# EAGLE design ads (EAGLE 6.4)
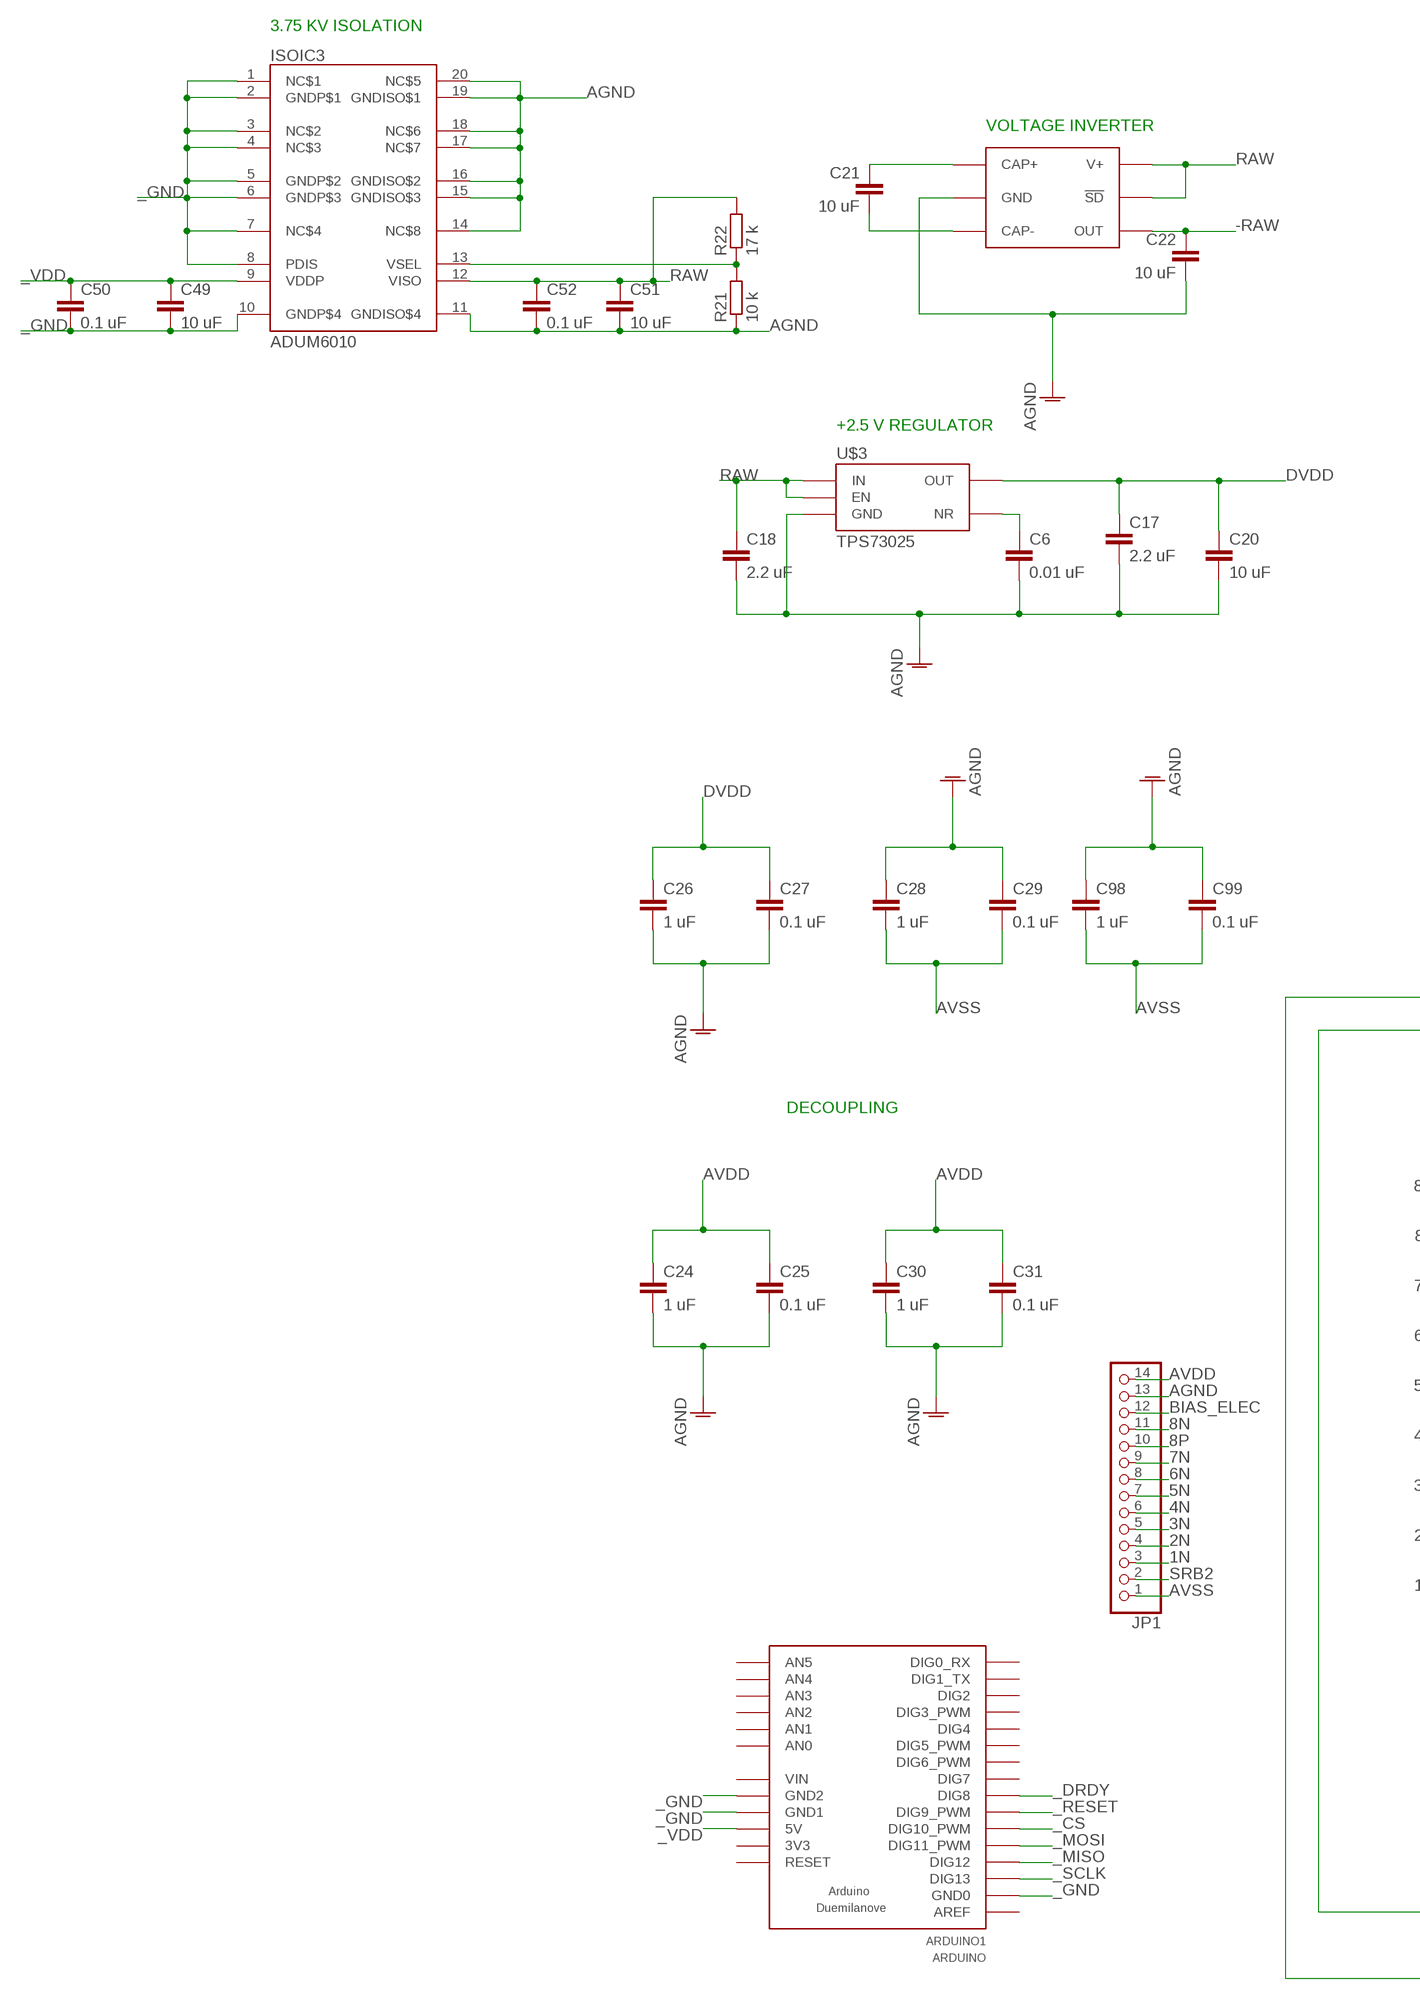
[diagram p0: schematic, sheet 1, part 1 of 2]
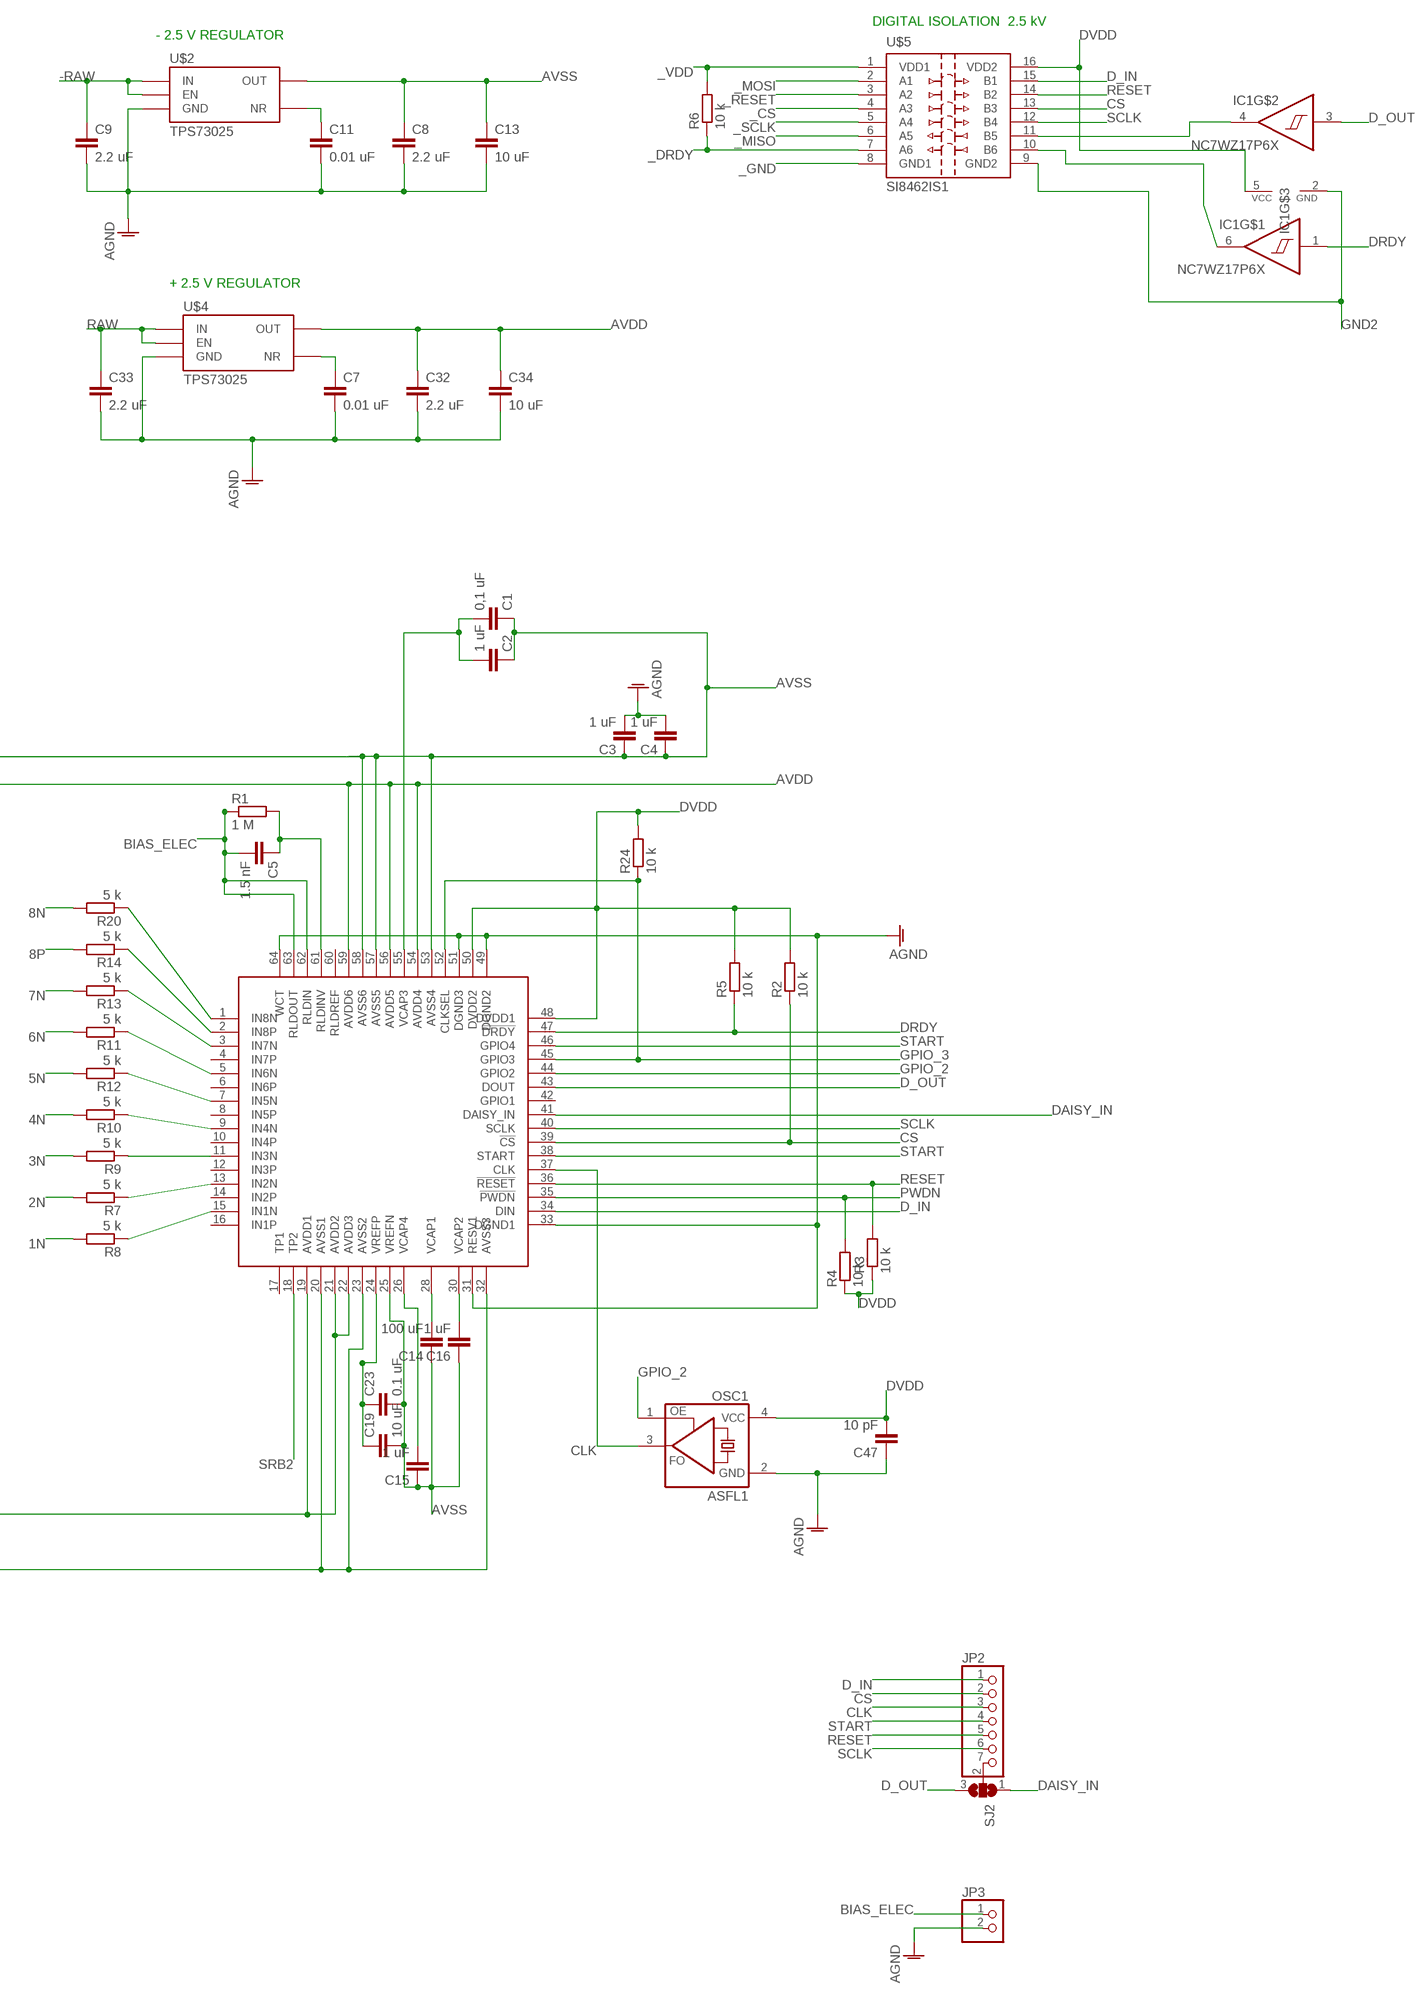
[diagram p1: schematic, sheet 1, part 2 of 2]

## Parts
ARDUINO1  ARDUINO  [ARDUINO]
C1  0,1 uF  C-EUC0603  [C0603]
C2  1 uF  C-EUC0603  [C0603]
C3  1 uF  C-EUC0603  [C0603]
C4  1 uF  C-EUC0603  [C0603]
C5  1.5 nF  C-EUC0603  [C0603]
C6  0.01 uF  C-EUC0603  [C0603]
C7  0.01 uF  C-EUC0603  [C0603]
C8  2.2 uF  C-EUC0603  [C0603]
C9  2.2 uF  C-EUC0603  [C0603]
C11  0.01 uF  C-EUC0603  [C0603]
C13  10 uF  C-EUC0603  [C0603]
C14  100 uF  C-EUC0603  [C0603]
C15  1 uF  C-EUC0603  [C0603]
C16  1 uF  C-EUC0603  [C0603]
C17  2.2 uF  C-EUC0603  [C0603]
C18  2.2 uF  C-EUC0603  [C0603]
C19  10 uF  C-EUC0603  [C0603]
C20  10 uF  C-EUC0603  [C0603]
C21  10 uF  C-EUC0603  [C0603]
C22  10 uF  C-EUC0603  [C0603]
C23  0.1 uF  C-EUC0603  [C0603]
C24  1 uF  C-EUC0603  [C0603]
C25  0.1 uF  C-EUC0603  [C0603]
C26  1 uF  C-EUC0603  [C0603]
C27  0.1 uF  C-EUC0603  [C0603]
C28  1 uF  C-EUC0603  [C0603]
C29  0.1 uF  C-EUC0603  [C0603]
C30  1 uF  C-EUC0603  [C0603]
C31  0.1 uF  C-EUC0603  [C0603]
C32  2.2 uF  C-EUC0603  [C0603]
C33  2.2 uF  C-EUC0603  [C0603]
C34  10 uF  C-EUC0603  [C0603]
C47  10 pF  C-EUC0603  [C0603]
C49  10 uF  C-EUC0603  [C0603]
C50  0.1 uF  C-EUC0603  [C0603]
C51  10 uF  C-EUC0603  [C0603]
C52  0.1 uF  C-EUC0603  [C0603]
C98  1 uF  C-EUC0603  [C0603]
C99  0.1 uF  C-EUC0603  [C0603]
IC1  NC7WZ17P6X  [SOT65P210X110-6AN_SC88_SC70-6]
ISOIC3  ADUM6010  [SSOP20]
JP1  PINHD-1X14/90  [1X14/90]
JP2  PINHD-1X7  [1X07]
JP3  PINHD-1X2  [1X02]
OSC1  ASFL1  [ASF]
R1  1 M  R-EU_R0603  [R0603]
R2  10 k  R-EU_R0603  [R0603]
R3  10 k  R-EU_R0603  [R0603]
R4  10 k  R-EU_R0603  [R0603]
R5  10 k  R-EU_R0603  [R0603]
R6  10 k  R-EU_R0603  [R0603]
R7  5 k  R-EU_R0603  [R0603]
R8  5 k  R-EU_R0603  [R0603]
R9  5 k  R-EU_R0603  [R0603]
R10  5 k  R-EU_R0603  [R0603]
R11  5 k  R-EU_R0603  [R0603]
R12  5 k  R-EU_R0603  [R0603]
R13  5 k  R-EU_R0603  [R0603]
R14  5 k  R-EU_R0603  [R0603]
R20  5 k  R-EU_R0603  [R0603]
R21  10 k  R-EU_R0603  [R0603]
R22  17 k  R-EU_R0603  [R0603]
R24  10 k  R-EU_R0603  [R0603]
SJ2  SJ2W  [SJ_2]
SOT-23-6  LM2664  [SOT23-6]
U$1  ADS1298-TQFP64  [TQFP64-10X10]
U$2  TPS73025  [SOT23-5L]
U$3  TPS73025  [SOT23-5L]
U$4  TPS73025  [SOT23-5L]
U$5  SI8462IS1  [SO16]

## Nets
1N: JP1.3 R8.2
2N: JP1.4 R7.2
3N: JP1.5 R9.2
4N: JP1.6 R10.2
5N: JP1.7 R12.2
6N: JP1.8 R11.2
7N: JP1.9 R13.2
8N: JP1.11 R20.2
8P: JP1.10 R14.2
-RAW: C9.1 C22.1 SOT-23-6.2(OUT) U$2.1(IN) U$2.3(EN)
_CS: ARDUINO1.D_10(DIG10_PWM) U$5.4(A3)
_DRDY: ARDUINO1.D_8(DIG8) R6.1 U$5.7(A6)
_GND: ARDUINO1.GND0 ARDUINO1.GND1 ARDUINO1.GND2 C49.2 C50.2 ISOIC3.1(NC$1) ISOIC3.2(GNDP$1) ISOIC3.3(NC$2) ISOIC3.4(NC$3) ISOIC3.5(GNDP$2) ISOIC3.6(GNDP$3) ISOIC3.7(NC$4) ISOIC3.8(PDIS) ISOIC3.10(GNDP$4) U$5.8(GND1)
_MISO: ARDUINO1.D_12(DIG12) U$5.6(A5)
_MOSI: ARDUINO1.D_11(DIG11_PWM) U$5.2(A1)
_RESET: ARDUINO1.D_9(DIG9_PWM) U$5.3(A2)
_SCLK: ARDUINO1.D_13(DIG13) U$5.5(A4)
_VDD: ARDUINO1.5V C49.1 C50.1 ISOIC3.9(VDDP) R6.2 U$5.1(VDD1)
AGND: C3.2 C4.2 C6.2 C7.2 C8.2 C9.2 C11.2 C13.2 C17.2 C18.2 C20.2 C22.2 C24.2 C25.2 C26.2 C27.2 C28.1 C29.1 C30.2 C31.2 C32.2 C33.2 C34.2 C47.1 C51.2 C52.2 C98.1 C99.1 ISOIC3.11(GNDISO$4) ISOIC3.14(NC$8) ISOIC3.15(GNDISO$3) ISOIC3.16(GNDISO$2) ISOIC3.17(NC$7) ISOIC3.18(NC$6) ISOIC3.19(GNDISO$1) ISOIC3.20(NC$5) JP1.13 JP3.2 OSC1.2(GND) R21.1 SOT-23-6.1(GND) U$1.31(RESV1) U$1.33(DGND1) U$1.49(DGND2) U$1.51(DGND3) U$1.64(WCT) U$2.2(GND) U$3.2(GND) U$4.2(GND)
AVDD: C24.1 C25.1 C30.1 C31.1 C32.1 C34.1 JP1.14 U$1.19(AVDD1) U$1.21(AVDD2) U$1.22(AVDD3) U$1.54(AVDD4) U$1.56(AVDD5) U$1.59(AVDD6) U$4.5(OUT)
AVSS: C1.1 C2.1 C3.1 C4.1 C8.1 C13.1 C14.1 C15.1 C16.1 C19.2 C23.2 C28.2 C29.2 C98.2 C99.2 JP1.1 U$1.20(AVSS1) U$1.23(AVSS2) U$1.25(VREFN) U$1.32(AVSS3) U$1.53(AVSS4) U$1.57(AVSS5) U$1.58(AVSS6) U$2.5(OUT)
BIAS_ELEC: C5.2 JP1.12 JP3.1 R1.1 U$1.62(RLDIN) U$1.63(RLDOUT)
CLK: JP2.3 OSC1.3(FO) U$1.37(CLK)
CS: JP2.2 R2.1 U$1.39(!CS) U$5.13(B3)
D_IN: JP2.1 U$1.34(DIN) U$5.15(B1)
D_OUT: IC1.3(I) SJ2.3 U$1.43(DOUT)
DAISY_IN: SJ2.1 U$1.41(DAISY_IN)
DRDY: IC1.1(I) R5.1 U$1.47(!DRDY)
DVDD: C17.1 C20.1 C26.1 C27.1 C47.2 IC1.5(VCC) OSC1.4(VCC) R2.2 R3.1 R4.1 R5.2 R24.2 U$1.48(DVDD1) U$1.50(DVDD2) U$3.5(OUT) U$5.16(VDD2)
GND2: IC1.2(GND) U$5.9(GND2)
GPIO_2: OSC1.1(OE) U$1.44(GPIO2)
GPIO_3: R24.1 U$1.45(GPIO3) U$1.52(CLKSEL)
IN1P: R8.1 U$1.15(IN1N)
IN2P: R7.1 U$1.13(IN2N)
IN3P: R9.1 U$1.11(IN3N)
IN4P: R10.1 U$1.9(IN4N)
IN5P: R12.1 U$1.7(IN5N)
N$1: JP2.7 SJ2.2
N$2: C11.1 U$2.4(NR)
N$3: C21.1 SOT-23-6.6(CAP+)
N$4: C14.2 U$1.28(VCAP1)
N$5: C16.2 U$1.30(VCAP2)
N$6: C1.2 C2.2 U$1.55(VCAP3)
N$7: C21.2 SOT-23-6.3(CAP-)
N$8: IC1.4(O) U$5.11(B5)
N$9: C19.1 C23.1 U$1.24(VREFP)
N$10: IC1.6(O) U$5.10(B6)
N$11: C5.1 R1.2 U$1.61(RLDINV)
N$12: C15.2 U$1.26(VCAP4)
N$13: C6.1 U$3.4(NR)
N$14: ISOIC3.13(VSEL) R21.2 R22.1
N$15: C7.1 U$4.4(NR)
N$16: R11.1 U$1.5(IN6N)
N$17: R13.1 U$1.3(IN7N)
N$19: R20.1 U$1.1(IN8N)
N$20: R14.1 U$1.2(IN8P)
PWDN: R4.2 U$1.35(!PWDN)
RAW: C18.1 C33.1 C51.1 C52.1 ISOIC3.12(VISO) R22.2 SOT-23-6.4(!SD) SOT-23-6.5(V+) U$3.1(IN) U$3.3(EN) U$4.1(IN) U$4.3(EN)
RESET: JP2.5 R3.2 U$1.36(!RESET) U$5.14(B2)
SCLK: JP2.6 U$1.40(SCLK) U$5.12(B4)
SRB2: JP1.2 U$1.18(TP2)
START: JP2.4 U$1.38(START) U$1.46(GPIO4)
Unconnected: ARDUINO1.3V3 ARDUINO1.A_0(AN0) ARDUINO1.A_1(AN1) ARDUINO1.A_2(AN2) ARDUINO1.A_3(AN3) ARDUINO1.A_4(AN4) ARDUINO1.A_5(AN5) ARDUINO1.AREF ARDUINO1.D_0(DIG0_RX) ARDUINO1.D_1(DIG1_TX) ARDUINO1.D_2(DIG2) ARDUINO1.D_3(DIG3_PWM) ARDUINO1.D_4(DIG4) ARDUINO1.D_5(DIG5_PWM) ARDUINO1.D_6(DIG6_PWM) ARDUINO1.D_7(DIG7) ARDUINO1.RESET U$1.4(IN7P) U$1.6(IN6P) U$1.8(IN5P) U$1.10(IN4P) U$1.12(IN3P) U$1.14(IN2P) U$1.16(IN1P) U$1.17(TP1) U$1.42(GPIO1) U$1.60(RLDREF)

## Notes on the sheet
- 3.75 KV ISOLATION
- DIGITAL ISOLATION  2.5 kV
- VOLTAGE INVERTER | - 2.5 V REGULATOR
- +2.5 V REGULATOR | + 2.5 V REGULATOR
- DECOUPLING

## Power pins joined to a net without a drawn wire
VIN: ARDUINO1.VIN

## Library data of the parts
ARDUINO1 = dp_devices:ARDUINO
C1-C9 C11 C13-C34 C47 C49-C52 C98 C99 = rcl:C-EU: CAPACITOR, European symbol
IC1 = fairchild-tinylogic:NC7W*17
ISOIC3 = SparkysWidgets:ADUM6010: ADUM6010 ISO DC-DC power uModule AD iCoupler based tech, dc-dc converter. Useful for galvanically isolating supplies accepts wide inpute range and outputs regulated 3v-5.v5@150mA
JP1 = pinhead:PINHD-1X14: PIN HEADER
JP2 = pinhead:PINHD-1X7: PIN HEADER
JP3 = pinhead:PINHD-1X2: PIN HEADER
OSC1 = crystal:ASF*: CRYSTAL CLOCK OSCILLATORS 5.0 Vdc or 3.3 Vdc - LOW PROFILE ULTRA MINIATURE CERAMIC SURFACE MOUNT Source: http://www.abracon.com/Oscillators/asf1-L-L1.pdf; MF: Abracon Corporation; MPN: ASFL1-125.000MHZ-EC-T; OC_FARNELL: 1838931; OC_NEWARK: 19M1882
R1-R14 R20-R22 R24 = rcl:R-EU_: RESISTOR, European symbol
SJ2 = jumper:SJ2W: SMD solder JUMPER
SOT-23-6 = lm2664:LM2664
U$1 = ads1298:ADS1298
U$2-U$4 = texas-instruments:TPS73025
U$5 = silicon-labs:SI8462: Si8462 6 Channel (4/2) Digital Isolator Silicon Labs Si84xx ISOpro digital isolator series. The Si84xx ISOpro digital isolators provide low power galvanic isolation for digital signals. They come in speeds of 1Mbps and 150Mbps, and isolation ratings of 1KV, 2.5KV and 5KV. The independent sides use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

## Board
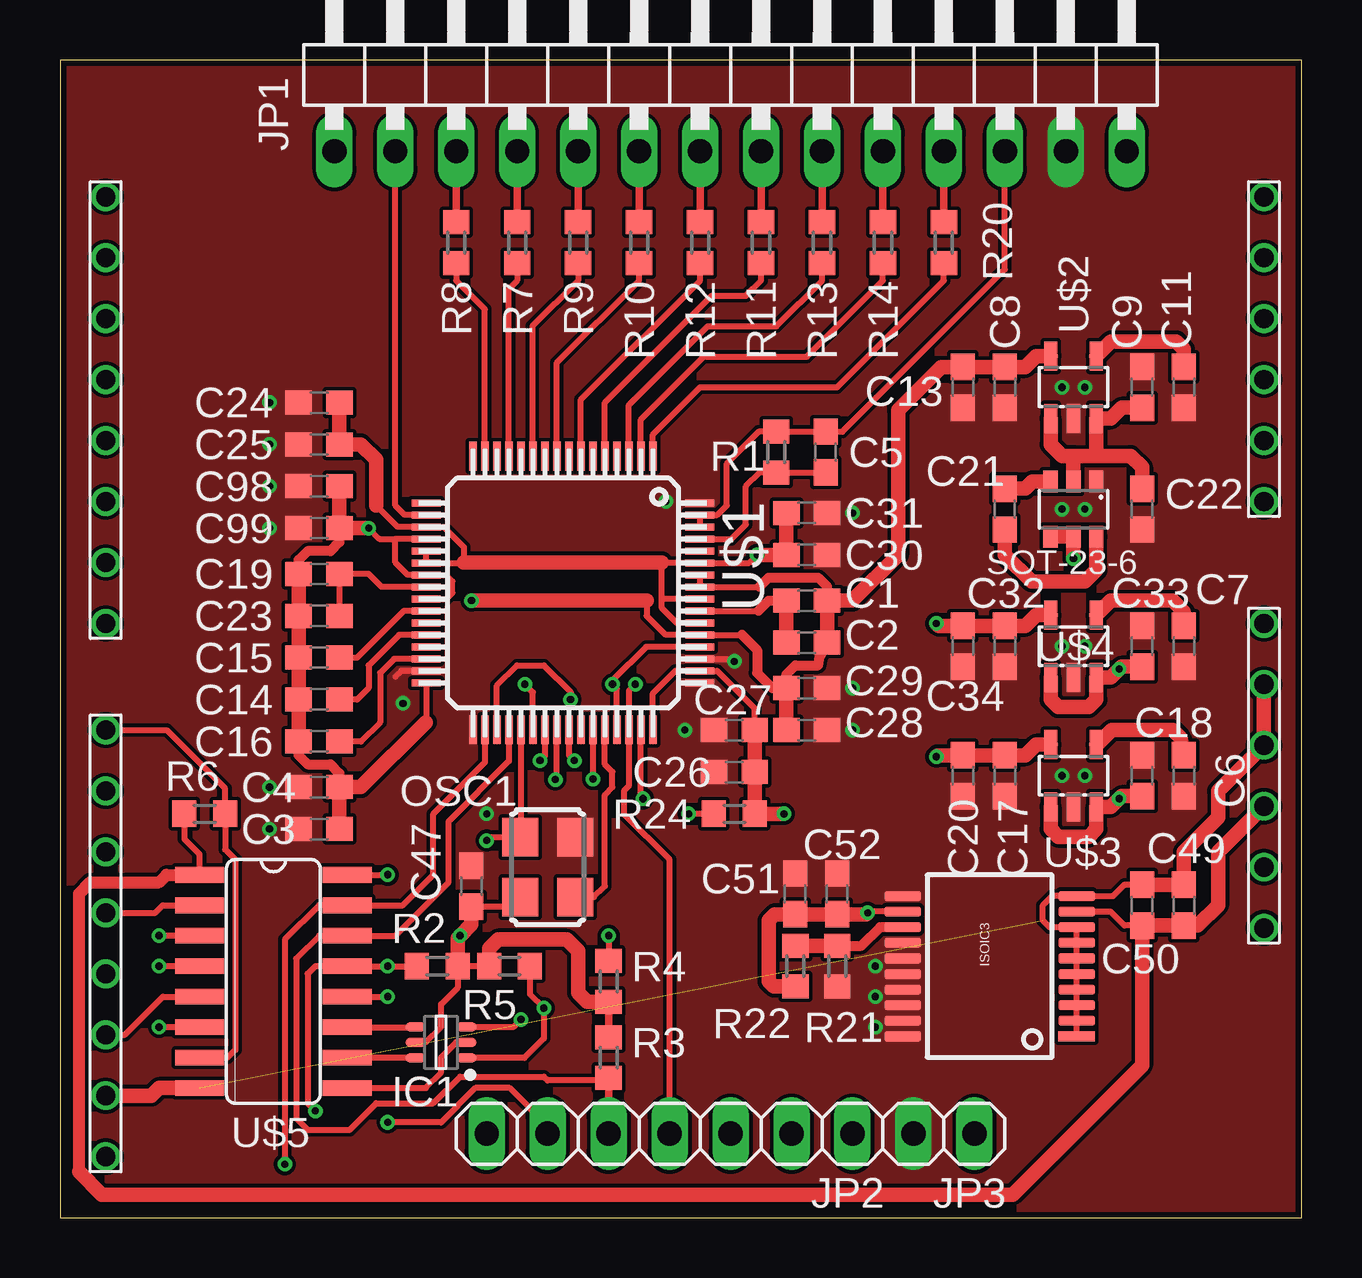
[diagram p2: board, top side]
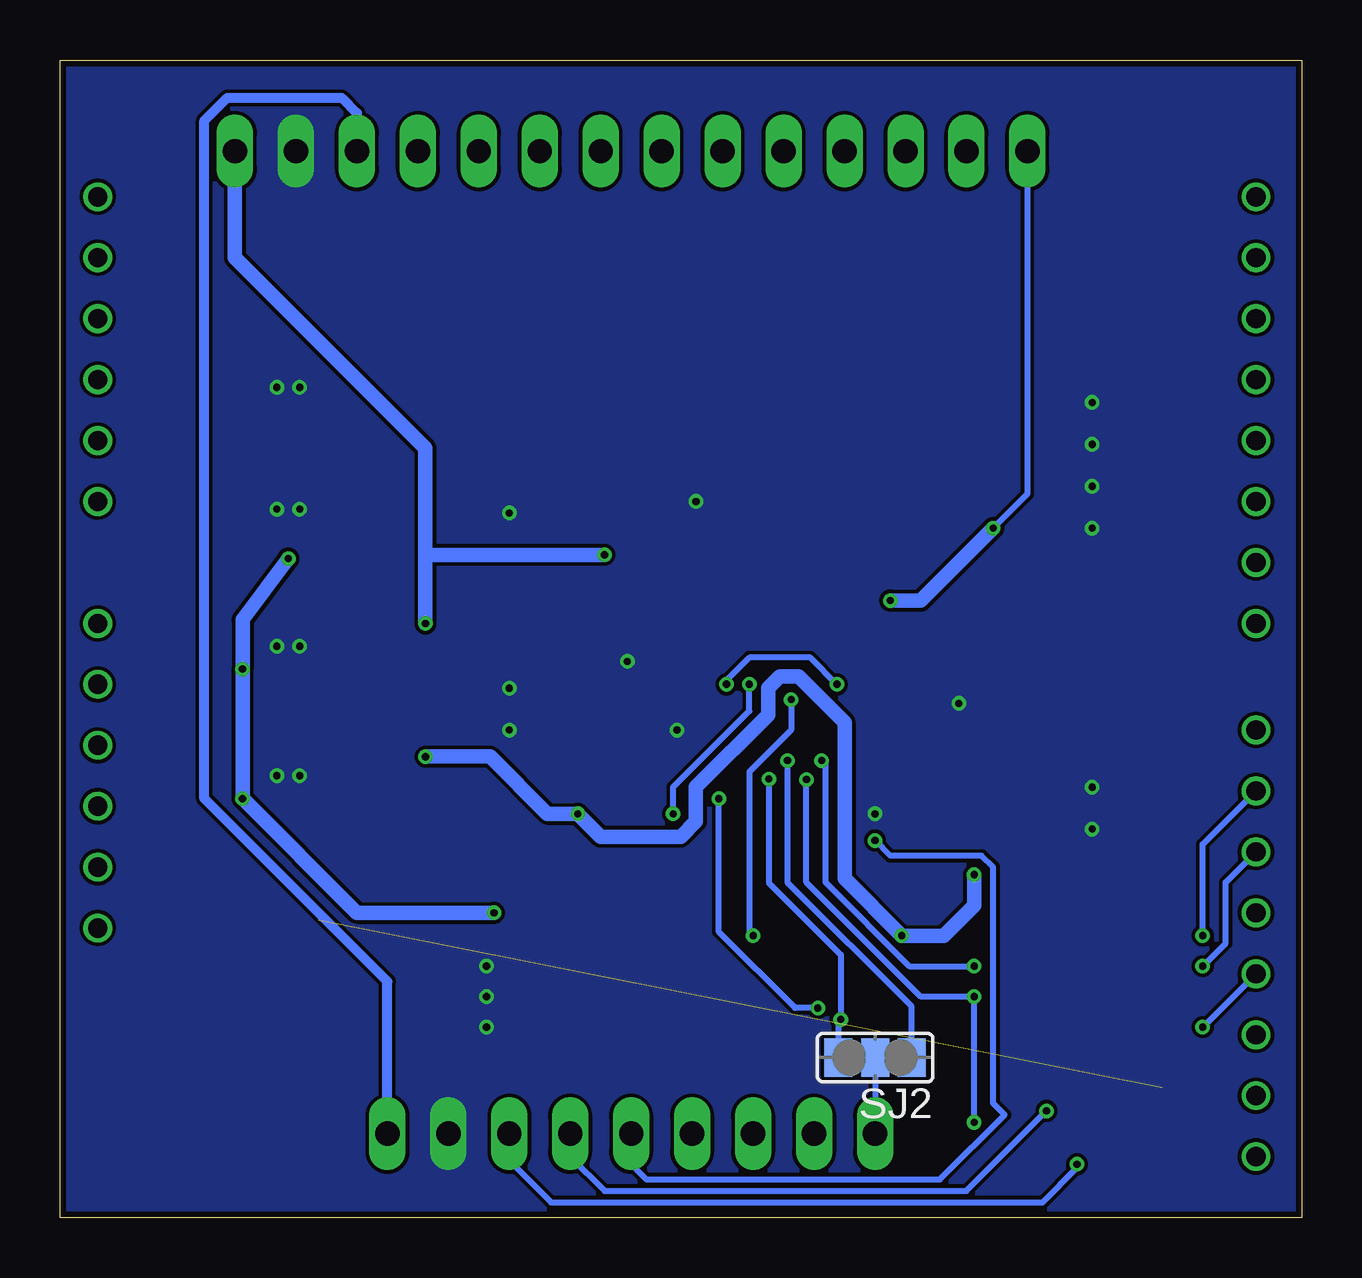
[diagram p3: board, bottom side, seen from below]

Size 51.74 x 48.25 mm. Coordinates in mm from the lower left corner, seen from the top.
Outline: 0,0 51.74,0 51.74,48.25 0,48.25 0,0
Copper layers (1*2*15*16): Top 0.035mm / dielectric 0.2mm / layer 2 0.0175mm / dielectric 1.1mm / layer 15 0.0175mm / dielectric 0.2mm / Bottom 0.035mm
Design rules "SeeedStudio_DRU_no_angle_20130527": minimum track width 6mil, minimum drill 12mil, track to track 6mil, track to pad 6mil, pad to pad 6mil, via to via 6mil, smd to smd 0mil, copper to edge 10mil, drill to drill 10mil, minimum pad ring 6mil, minimum via ring 6mil, stop-mask expansion 2mil, vias tented up to drill 25mil, thermal gap 10mil

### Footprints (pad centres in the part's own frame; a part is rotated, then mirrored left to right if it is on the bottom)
ARDUINO = drill 0.8: 3V3 25.4,-12.7; 5V 25.4,-10.16; A_0 25.4,2.54; A_1 25.4,5.08; A_2 25.4,7.62; A_3 25.4,10.16; A_4 25.4,12.7; A_5 25.4,15.24; AREF -22.86,-24.765; D_0 -22.86,15.24; D_1 -22.86,12.7; D_2 -22.86,10.16; D_3 -22.86,7.62; D_4 -22.86,5.08; D_5 -22.86,2.54; D_6 -22.86,0; D_7 -22.86,-2.54; D_8 -22.86,-6.985; D_9 -22.86,-9.525; D_10 -22.86,-12.065; D_11 -22.86,-14.605; D_12 -22.86,-17.145; D_13 -22.86,-19.685; GND0 -22.86,-22.225; GND1 25.4,-7.62; GND2 25.4,-5.08; RESET 25.4,-15.24; VIN 25.4,-2.54
C0603 = smd 1.1 x 1: 1 -0.85,0; 2 0.85,0
SOT65P210X110-6AN_SC88_SC70-6 = smd 0.85 x 0.4: 1 -1.05,0.65; 2 -1.05,0; 3 -1.05,-0.65; 4 1.05,-0.65; 5 1.05,0; 6 1.05,0.65
SSOP20 = smd 0.419 x 1.524: 1 -2.925,-3.625; 2 -2.275,-3.625; 3 -1.625,-3.625; 4 -0.975,-3.625; 5 -0.325,-3.625; 6 0.325,-3.625; 7 0.975,-3.625; 8 1.625,-3.625; 9 2.275,-3.625; 10 2.925,-3.625; 11 2.925,3.625; 12 2.275,3.625; 13 1.625,3.625; 14 0.975,3.625; 15 0.325,3.625; 16 -0.325,3.625; 17 -0.975,3.625; 18 -1.625,3.625; 19 -2.275,3.625; 20 -2.925,3.625
1X14/90 = drill 1.016 long: 1 -16.51,-3.81; 2 -13.97,-3.81; 3 -11.43,-3.81; 4 -8.89,-3.81; 5 -6.35,-3.81; 6 -3.81,-3.81; 7 -1.27,-3.81; 8 1.27,-3.81; 9 3.81,-3.81; 10 6.35,-3.81; 11 8.89,-3.81; 12 11.43,-3.81; 13 13.97,-3.81; 14 16.51,-3.81
1X07 = drill 1.016 long: 1 -7.62,0; 2 -5.08,0; 3 -2.54,0; 4 0,0; 5 2.54,0; 6 5.08,0; 7 7.62,0
1X02 = drill 1.016 long: 1 -1.27,0; 2 1.27,0
ASF = smd 1.6 x 1.5: 1 -1.25,-1.15; 2 1.25,-1.15; 3 1.25,1.15; 4 -1.25,1.15
R0603 = smd 1 x 1.1: 1 -0.85,0; 2 0.85,0
SJ_2 = smd 1.168 x 1.6: 1 -1.524,0; 2 0,0; 3 1.524,0
SOT23-6 = smd 0.6 x 0.9: 1 -0.95,-1.15; 2 0,-1.15; 3 0.95,-1.15; 4 0.95,1.15; 5 0,1.15; 6 -0.95,1.15
TQFP64-10X10 = smd 1.2 x 0.3: 1 -5.7,3.75; 2 -5.7,3.25; 3 -5.7,2.75; 4 -5.7,2.25; 5 -5.7,1.75; 6 -5.7,1.25; 7 -5.7,0.75; 8 -5.7,0.25; 9 -5.7,-0.25; 10 -5.7,-0.75; 11 -5.7,-1.25; 12 -5.7,-1.75; 13 -5.7,-2.25; 14 -5.7,-2.75; 15 -5.7,-3.25; 16 -5.7,-3.75; 33 5.7,-3.75; 34 5.7,-3.25; 35 5.7,-2.75; 36 5.7,-2.25; 37 5.7,-1.75; 38 5.7,-1.25; 39 5.7,-0.75; 40 5.7,-0.25; 41 5.7,0.25; 42 5.7,0.75; 43 5.7,1.25; 44 5.7,1.75; 45 5.7,2.25; 46 5.7,2.75; 47 5.7,3.25; 48 5.7,3.75 | smd 0.3 x 1.2: 17 -3.75,-5.7; 18 -3.25,-5.7; 19 -2.75,-5.7; 20 -2.25,-5.7; 21 -1.75,-5.7; 22 -1.25,-5.7; 23 -0.75,-5.7; 24 -0.25,-5.7; 25 0.25,-5.7; 26 0.75,-5.7; 27 1.25,-5.7; 28 1.75,-5.7; 29 2.25,-5.7; 30 2.75,-5.7; 31 3.25,-5.7; 32 3.75,-5.7; 49 3.75,5.7; 50 3.25,5.7; 51 2.75,5.7; 52 2.25,5.7; 53 1.75,5.7; 54 1.25,5.7; 55 0.75,5.7; 56 0.25,5.7; 57 -0.25,5.7; 58 -0.75,5.7; 59 -1.25,5.7; 60 -1.75,5.7; 61 -2.25,5.7; 62 -2.75,5.7; 63 -3.25,5.7; 64 -3.75,5.7
SOT23-5L = smd 0.55 x 1.2: 1 -0.95,-1.3; 2 0,-1.3; 3 0.95,-1.3; 4 0.95,1.3; 5 -0.95,1.3
SO16 = smd 0.66 x 2.032: 1 -4.445,-3.073; 2 -3.175,-3.073; 3 -1.905,-3.073; 4 -0.635,-3.073; 5 0.635,-3.073; 6 1.905,-3.073; 7 3.175,-3.073; 8 4.445,-3.073; 9 4.445,3.073; 10 3.175,3.073; 11 1.905,3.073; 12 0.635,3.073; 13 -0.635,3.073; 14 -1.905,3.073; 15 -3.175,3.073; 16 -4.445,3.073

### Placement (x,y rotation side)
ARDUINO1  24.77,27.3 0 top
C1  31.11,25.72 180 top
C2  31.11,23.97 180 top
C3  10.79,16.19 180 top
C4  10.79,17.94 180 top
C5  31.91,31.91 90 top
C6  46.83,18.41 270 top
C7  46.83,23.81 270 top
C8  39.37,34.61 270 top
C9  45.09,34.61 90 top
C11  46.83,34.61 270 top
C13  37.62,34.61 270 top
C14  10.79,21.59 0 top
C15  10.79,23.34 0 top
C16  10.79,19.84 0 top
C17  39.37,18.41 270 top
C18  45.09,18.41 90 top
C19  10.79,26.83 180 top
C20  37.62,18.41 270 top
C21  39.37,29.53 90 top
C22  45.09,29.53 270 top
C23  10.79,25.08 180 top
C24  10.79,33.97 180 top
C25  10.79,32.23 180 top
C26  28.1,18.57 180 top
C27  28.1,20.32 180 top
C28  31.11,20.32 180 top
C29  31.11,22.07 180 top
C30  31.11,27.62 0 top
C31  31.11,29.37 0 top
C32  39.37,23.81 270 top
C33  45.09,23.81 90 top
C34  37.62,23.81 270 top
C47  17.14,13.81 270 top
C49  46.83,13.02 90 top
C50  45.09,13.02 90 top
C51  30.64,13.49 90 top
C52  32.38,13.49 90 top
C98  10.79,30.48 0 top
C99  10.79,28.73 0 top
IC1  15.88,7.3 180 top
ISOIC3  38.73,10.48 90 top
JP1  27.94,48.26 0 top
JP2  25.4,3.49 180 top
JP3  36.83,3.49 180 top
OSC1  20.32,14.61 90 top
R1  29.84,31.91 270 top
R2  15.72,10.48 0 top
R3  22.86,6.67 270 top
R4  22.86,9.84 90 top
R5  18.73,10.48 180 top
R6  6.03,16.83 180 top
R7  19.05,40.64 90 top
R8  16.51,40.64 90 top
R9  21.59,40.64 90 top
R10  24.13,40.64 90 top
R11  29.21,40.64 90 top
R12  26.67,40.64 90 top
R13  31.75,40.64 90 top
R14  34.29,40.64 90 top
R20  36.83,40.64 90 top
R21  32.38,10.48 90 top
R22  30.64,10.48 270 top
R24  28.1,16.83 0 top
SJ2  17.78,6.67 180 bottom
SOT-23-6  42.23,29.53 180 top
U$1  20.95,26.04 270 top
U$2  42.23,34.61 0 top
U$3  42.23,18.41 0 top
U$4  42.23,23.81 0 top
U$5  8.89,9.84 270 top

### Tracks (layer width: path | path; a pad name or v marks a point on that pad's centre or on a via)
1N
  Top 0.305: JP1.3 R8.2
2N
  Top 0.305: R7.2 JP1.4
3N
  Top 0.305: R9.2 JP1.5
4N
  Top 0.305: R10.2 JP1.6
5N
  Top 0.305: R12.2 JP1.7
6N
  Top 0.305: R11.2 JP1.8
7N
  Top 0.305: R13.2 JP1.9
8N
  Top 0.305: R20.2 JP1.11
8P
  Top 0.305: R14.2 JP1.10
-RAW
  Top 0.61: 43.18,31.75 44.61,31.75 45.09,31.27 C22.1 | 43.18,31.75 U$2.3 43.78,33.31 44.23,33.76 C9.1 | U$2.1 41.28,32.22 41.75,31.75 42.23,31.75 | 42.23,31.75 43.18,31.75 | SOT-23-6.2 42.23,31.75
_CS  (via drill 0.3)
  Top 0.254: U$5.4 v4.13,10.48
  Bottom 0.254: v4.13,10.48 3.17,11.43 3.17,13.97 ARDUINO1.D_10
_DRDY
  Top 0.254: U$5.7 6.99,6.67 7.3,6.99 7.3,14.92 6.88,15.34 R6.1 6.88,17.88 4.45,20.32 ARDUINO1.D_8
_GND  (1 unrouted)
  Top 0.254: C50.2 44.35,13.87 43.88,13.4 ISOIC3.10 41.34,13.4 40.96,13.02 40.96,12.38 41.24,12.1 ISOIC3.8 ISOIC3.7 ISOIC3.6 ISOIC3.5 ISOIC3.4 ISOIC3.3 ISOIC3.2 ISOIC3.1
  Top 0.61: C50.2 C49.2 46.83,15.24 48.26,16.67 48.26,17.78 ARDUINO1.GND1 ARDUINO1.GND2 | U$5.8 4.13,5.4 3.81,5.08 ARDUINO1.GND0
_MISO  (via drill 0.3)
  Top 0.254: U$5.6 v4.13,7.94
  Bottom 0.254: ARDUINO1.D_12 v4.13,7.94
_MOSI
  Top 0.254: ARDUINO1.D_11 3.97,12.7 4.29,13.02 U$5.2
_RESET  (via drill 0.3)
  Top 0.254: U$5.3 v4.13,11.75
  Bottom 0.254: v4.13,11.75 4.13,15.56 ARDUINO1.D_9
_SCLK
  Top 0.254: ARDUINO1.D_13 2.7,7.62 4.29,9.21 U$5.5
_VDD
  Top 0.254: U$5.1 5.82,15.14 5.18,15.77 R6.2 | ISOIC3.9 43.76,12.75 44.35,12.17 C50.1
  Top 0.508: 0.79,1.91 0.79,13.49 1.27,13.97 4.13,13.97 4.45,14.29 U$5.1
  Top 0.61: ARDUINO1.5V 48.26,15.24 48.26,13.02 47.41,12.17 C49.1 C50.1 45.09,6.35 39.69,0.95 1.75,0.95 0.79,1.91
AGND  (via drill 0.3)
  Top 0.254: 15.08,22.79 U$1.31 14.21,22.79 13.97,22.54 | U$1.51 27.99,23.29 v28.1,23.18
  other vias: 33.02,22.07 33.02,20.32 42.7,23.81 41.75,23.81 41.75,29.53 42.7,29.53 42.7,34.61 41.75,34.61 42.7,18.41 41.75,18.41 14.29,21.43 8.73,17.94 8.73,16.19 8.73,28.73 8.73,30.48 8.73,32.23 8.73,33.97 25.24,29.84 26.04,20.32 17.78,16.83 33.02,29.37 33.97,10.48 33.97,9.21 33.97,7.94
  pour Top (no thermals): 0,0 52.07,0 52.07,48.26 0,48.26
  pour Bottom (no thermals): 0,0 51.75,0 51.75,48.26 0,48.26
AVDD  (via drill 0.3)
  Top 0.254: U$1.21 U$1.22 16.81,27.29 16.83,27.3 16.83,27.94 15.98,28.79 U$1.19 14.08,28.79 13.18,29.69 | U$1.54 25.7,24.79 25.08,25.4 25.08,25.72 | 25.08,25.72 25.08,27.3 25.1,27.29 U$1.59 28.71,27.29 v29.05,27.62 | U$1.56 25.15,25.79 25.08,25.72
  Top 0.61: 25.08,27.3 16.83,27.3 | C24.1 C25.1 12.54,32.23 13.18,31.59 13.18,29.69 | C31.1 C30.1 v29.05,27.62 | U$4.5 40.67,25.11 40.22,24.66 C32.1 C34.1 36.62,24.66 v36.51,24.77
  Bottom 0.61: JP1.14 44.45,40.01 36.51,32.07 36.51,27.62 | 36.51,27.62 v36.51,24.77 | v29.05,27.62 36.51,27.62
AVSS  (via drill 0.3)
  Top 0.254: U$1.20 13.97,28.29 | 24.45,25.72 24.45,25.08 25.25,24.29 U$1.53 28.42,24.29 | 13.97,28.29 13.97,27.3 14.49,26.79 U$1.23 16.08,26.79 16.35,26.51 16.35,26.04 16.1,25.79 U$1.25 | U$1.58 U$1.57 29.14,26.29 | U$1.32 15.26,20.65 15.24,20.64 | v12.86,28.73 13.31,28.29 13.97,28.29
  Top 0.406: C99.2 11.64,28.16 11.27,27.78 10.32,27.78 9.95,27.41 C19.2 | 28.42,24.29 29.05,23.65 29.05,22.7 29.69,22.07 C29.2 30.27,22.64 30.64,23.02 31.59,23.02 31.65,23.39 C2.1 | 29.14,26.29 29.53,26.67 31.59,26.67 31.96,26.3 C1.1 | C16.1 9.95,19.27 10.32,18.89 11.27,18.89 11.64,18.52 C4.1
  Top 0.61: v12.86,28.73 C99.2 C98.2 | C16.1 C14.1 C15.1 C23.2 C19.2 | 24.45,25.72 v17.14,25.72 | C29.2 C28.2 | C2.1 C1.1 33.02,25.72 34.92,27.62 34.92,33.66 36.73,35.46 C13.1 C8.1 40.22,35.46 40.67,35.91 U$2.5 | C3.1 C4.1 12.54,17.94 15.24,20.64
  Bottom 0.254: JP1.1 11.43,30.16 v12.86,28.73
  Bottom 0.61: v17.14,25.72 15.88,25.72 v12.86,28.73
BIAS_ELEC
  Top 0.254: U$1.62 U$1.63 27.38,29.29 27.78,29.69 27.78,31.43 29.11,32.76 R1.1 C5.2 32.6,32.76 39.37,39.53 JP1.12
  Bottom 0.406: JP3.1 38.1,9.84 45.72,17.46 45.72,45.72 44.77,46.67 40.01,46.67 39.37,46.04 JP1.12
CLK  (via drill 0.3)
  Top 0.254: U$1.37 19.2,15.89 OSC1.3 17.92,15.86 v17.78,15.72
  Bottom 0.254: JP2.3 27.94,2.22 27.3,1.59 15.08,1.59 12.38,4.29 12.86,4.76 12.86,14.61 13.34,15.08 17.14,15.08 v17.78,15.72
CS  (via drill 0.3)
  Top 0.254: R2.1 v13.65,10.48 U$5.13 10.64,10.48 10.32,10.16 10.32,4.76 v10.64,4.45 | U$1.39 20.2,19.25 v20,19.05
  Bottom 0.254: v13.65,10.48 16.35,10.48 19.84,13.97 19.84,18.89 v20,19.05 | JP2.2 30.48,2.54 29.05,1.11 13.97,1.11 v10.64,4.45
D_IN  (via drill 0.3)
  Top 0.254: U$1.34 17.7,18.98 15.56,16.83 15.56,14.29 14.29,13.02 U$5.15 10.79,13.02 9.37,11.59 v9.37,2.22
  Bottom 0.254: JP2.1 33.02,2.38 31.27,0.64 10.79,0.64 9.37,2.06 v9.37,2.22
D_OUT  (via drill 0.3)
  Top 0.254: U$1.43 v22.2,18.28 22.23,18.26 | IC1.3 18.91,7.95 v19.21,8.26
  Bottom 0.254: v22.2,18.28 22.2,13.95 19.21,10.95 v19.21,8.26 19.3,8.16 SJ2.3
DAISY_IN  (via drill 0.3)
  Top 0.254: U$1.41 21.2,19.28 v21.43,19.05
  Bottom 0.254: v21.43,19.05 21.43,13.97 16.26,8.79 SJ2.1
DRDY  (via drill 0.3)
  Top 0.254: R5.1 19.58,9.31 v20.16,8.73 20.16,7.46 19.35,6.65 IC1.1 | v24.29,17.46 24.2,17.54 U$1.47
  Bottom 0.254: v20.16,8.73 21.11,8.73 24.29,11.91 v24.29,17.46
DVDD  (via drill 0.3)
  Top 0.254: U$1.48 24.7,21.85 25.64,22.79 U$1.50 27.38,22.79 28.95,21.22 C27.1 | C47.2 18.78,12.96 OSC1.4 | IC1.5 15.24,7.3 15.88,7.94 15.88,8.89 16.57,9.58 R2.2 R5.2 | U$5.16 v13.65,14.29
  Top 0.305: R3.1 R4.1
  Top 0.61: U$3.5 40.67,19.71 40.22,19.27 C17.1 C20.1 36.57,19.27 v36.51,19.21 | R2.2 16.57,11.64 v16.67,11.75 17.14,12.22 C47.2 | v30.16,16.83 R24.2 C26.1 C27.1 | R4.1 21.96,8.99 21.59,9.37 21.59,11.11 21.11,11.59 18.26,11.59 17.88,11.21 R5.2
  Bottom 0.61: v36.51,19.21 33.81,19.21 31.43,16.83 v30.16,16.83 29.21,15.88 25.88,15.88 25.24,16.51 25.24,17.94 22.23,20.95 22.23,22.07 21.75,22.54 20.95,22.54 19.05,20.64 19.05,14.13 v16.67,11.75 14.92,11.75 13.65,13.02 v13.65,14.29
GND2
  Top 0.254: U$5.9 15.24,5.4 15.88,6.03 15.88,6.67 16.51,7.3 IC1.2
GPIO_2
  Top 0.254: OSC1.1 22.25,13.36 22.7,13.81 22.7,17.62 23.02,17.94 23.02,18.57 22.7,18.89 U$1.44
GPIO_3  (via drill 0.3)
  Top 0.254: U$1.52 24.42,23.79 23.02,22.38 v23.02,22.23 23.2,22.04 U$1.45 | R24.1 v26.19,16.83
  Bottom 0.254: v23.02,22.23 23.02,21.11 26.19,17.94 v26.19,16.83
IN1P
  Top 0.254: R8.1 16.51,39.05 17.7,37.86 U$1.15
IN2P
  Top 0.254: R7.1 19.05,39.05 18.7,38.71 U$1.13
IN3P
  Top 0.254: R9.1 21.59,39.05 19.68,37.15 19.68,31.75 U$1.11
IN4P
  Top 0.254: U$1.9 20.7,35.63 24.13,39.05 R10.1
IN5P
  Top 0.254: U$1.7 21.7,34.09 26.67,39.05 R12.1
  Top 0.305: 26.47,39.59 R12.1
N$1
  Bottom 0.254: SJ2.2 JP2.7
N$2
  Top 0.61: C11.1 46.83,36.2 46.51,36.51 43.78,36.51 U$2.4
N$3
  Top 0.61: C21.1 39.37,27.62 40.48,26.51 42.7,26.51 43.18,26.99 SOT-23-6.6
N$4
  Top 0.254: U$1.28 14.12,24.29 12.86,23.02 12.86,22.07 12.38,21.59 C14.2
N$5
  Top 0.254: U$1.30 13.92,23.29 13.34,22.7 13.34,20.64 12.54,19.84 C16.2
N$6
  Top 0.254: U$1.55 29.09,25.29
  Top 0.406: 29.09,25.29 29.53,25.72 C1.2
  Top 0.61: C1.2 C2.2
N$7
  Top 0.61: C21.2 40.22,30.38 40.52,30.68 SOT-23-6.3
N$8
  Top 0.254: U$5.11 14.81,7.94 IC1.4
N$9
  Top 0.254: U$1.24 13.4,26.29 12.86,26.83 C19.1 C23.1
N$10
  Top 0.254: U$5.10 14.81,6.67 IC1.6
N$11
  Top 0.254: U$1.61 27.97,28.29 28.57,28.89 28.57,30.48 29.15,31.06 R1.2 C5.1
N$12
  Top 0.254: C15.2 12.38,23.34 14.33,25.29 U$1.26
N$13
  Top 0.61: U$3.4 43.21,19.71 43.81,20.32 46.35,20.32 46.67,20 C6.1
N$14
  Top 0.406: ISOIC3.13 34.17,12.1 33.39,11.33 R21.2
  Top 0.61: R22.1 R21.2
N$15
  Top 0.61: U$4.4 43.78,25.72 46.35,25.72 46.83,25.24 C7.1
N$16
  Top 0.254: U$1.5 22.7,33.98 27.15,38.42 28.57,38.42 29.21,39.05 R11.1
N$17
  Top 0.254: U$1.3 23.7,33.87 26.99,37.15 29.84,37.15 31.75,39.05 R13.1
N$19
  Top 0.254: R20.1 36.83,39.05 32.38,34.61 26.67,34.61 24.7,32.64 U$1.1
N$20
  Top 0.254: U$1.2 24.2,33.25 26.83,35.88 31.11,35.88 34.29,39.05 R14.1
PWDN  (via drill 0.3)
  Top 0.254: U$1.35 18.2,22.17 19.05,23.02 20.16,23.02 21.27,21.91 v21.27,21.59 | v22.86,11.75 R4.2
  Bottom 0.254: v21.27,21.59 21.27,20.32 23.02,18.57 23.02,11.91 v22.86,11.75
RAW  (via drill 0.3)
  Top 0.254: ISOIC3.12 33.71,12.75 v33.66,12.7
  Top 0.61: C18.1 44.23,17.57 v44.13,17.46 43.78,17.11 U$3.3 43.18,16.19 42.86,15.88 41.59,15.88 41.28,16.19 U$3.1 | C33.1 44.23,22.96 v44.13,22.86 43.78,22.51 U$4.3 43.18,21.59 42.86,21.27 41.59,21.27 41.28,21.59 U$4.1 | SOT-23-6.4 SOT-23-6.5 v42.23,27.46 | v33.66,12.7 33.6,12.64 C52.1 C51.1 29.79,12.64 29.53,12.38 29.53,9.84 29.74,9.63 R22.2
  Bottom 0.61: v42.23,27.46 44.13,24.92 v44.13,22.86 v44.13,17.46 39.37,12.7 v33.66,12.7
RESET
  Top 0.254: U$1.36 18.7,19.02 16.19,16.51 16.19,13.97 13.97,11.75 U$5.14 10.79,11.75 9.84,10.79 9.84,4.13 10.32,3.65 12.06,3.65 13.18,4.76 15.56,4.76 16.67,5.87 20.16,5.87 20.32,5.71 22.76,5.71
  Top 0.305: JP2.5 R3.2 22.76,5.71
SCLK  (via drill 0.3)
  Top 0.254: U$5.12 v13.65,9.21 | v20.64,18.26 20.7,18.32 U$1.40 | JP2.6 20.32,3.81 18.73,5.4 17.3,5.4 15.88,3.97 v13.65,3.97
  Bottom 0.254: v20.64,18.26 20.64,13.97 15.88,9.21 v13.65,9.21 v13.65,3.97
SRB2
  Top 0.254: U$1.18 14.37,29.29 13.97,29.69 JP1.2
START  (via drill 0.3)
  Top 0.254: v23.97,22.23 23.7,21.96 U$1.46 23.7,17.99 23.5,17.78 23.5,16.83 25.4,14.92 JP2.4 | U$1.38 19.7,21.89 v19.37,22.23
  Bottom 0.254: v19.37,22.23 20.48,23.34 23.02,23.34 23.97,22.38 v23.97,22.23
